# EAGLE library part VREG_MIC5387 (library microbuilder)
MIC5387 - Triple Output Linear LDO Regulator 150ma Output on each LDO, 180mV Vf, 2.5-5.5V Input 3.3V, 1.8V, 1.2V - Digikey: 576-3689-1-ND
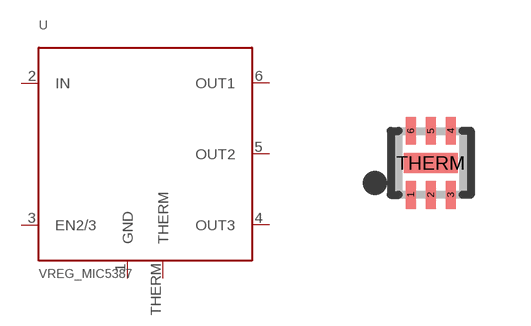
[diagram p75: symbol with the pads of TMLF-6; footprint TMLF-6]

Designator prefix U

## VREG_MIC5387  [TMLF-6]
1  GND
2  IN
3  EN2/3
4  OUT3
5  OUT2
6  OUT1
THERM  THERM

## Footprint TMLF-6 (pad centres in mm)
6-Pin 1.6mm x 1.6mm Thin MLF Source: http://www.micrel.com/_PDF/mic5387.pdf
smd 0.25 x 0.7: 1 -0.5,-0.8; 2 0,-0.8; 3 0.5,-0.8; 4 0.5,0.8; 5 0,0.8; 6 -0.5,0.8
smd 1.35 x 0.5: THERM 0,0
